ORGANIZATION_BLOCK MAIN:OB1
TITLE= Ciclo Automatico A+/A- per un cilindro a doppio effetto
// Simulatore: 04
// Versione: 1.0
// Data: 28/02/2002
//-------- Descrizione del Controllo --------------------------------
// L'esempio presenta il comando di un cilindro pneumatico a
// doppio effetto (A) mediante un'elettrovalvola 5/2 bistabile (1V1).
// Nel circuito è presente anche un'elettrovalvola del tipo 3/2
// monostabile (0V) che comanda la distribuzione dell'aria nel
// circuito.
// Sulle mandate di alimentazione del cilindro A sono presenti due
// strozzatori unidirezionali per la regolazione della velocità
// delle due corse (A+ e A-) del pistone.
// Un circuito di sicurezza esterno al PLC provvede, quando viene
// disttivato a far rientrare lo stelo del cilindro  nella posizione
// di riposo A- indipendentemente dalle uscite del PLC, che vengono
// resettate quandondo il pulsante SB1 (che simula l'intervento del
// circuito di sicurezza esterno) viene premuto.
// Per le segnalazioni è previste la lampade HL1 che indica
// la presenza dell'aria .
// Agli ingressi del PLC vengono inviati:
// 1)Il selettore SB6 per il comando di 0Y1 che fornisce l'aria
//   compressa al circuito elettropneumatico;
// 2)Il pulsante di arresto a fine ciclo SB3 (NC);
// 3)Il pulsante di inizio ciclo ripetitivo SB2;
// 4)Il pulsante di inizio ciclo non ripetitivo SB4;
// 5)I fine corsa magnetici a0 e a1 che controllano la posizione
//   del pistone rispettivamente in a- e a+;
// L'eventuale mancata eccitazione dell'elettrovalvola distributrice
// non consente l'avvio del ciclo ripetitivo.
//

BEGIN
NETWORK 1 //Comando alimentazione aria elettrovalvola 0V
//
LD I0.0
= Q0.0

NETWORK 2 //Comando Inizio ciclo
//
LD I0.4
O M0.0
A I0.5
A Q0.0
AN I0.3
= M0.0

NETWORK 3 //Comando EV. 1Y1 (uscita cilindro A+)
//
LD M0.0
O I0.6
A I0.1
= Q0.1

NETWORK 4 //Comando EV. 1Y2  (rientro cilindro A-)
//
LD I0.2
= Q0.2

NETWORK 5 //Segnalazione presenza aria compressa
//
LD Q0.0
= Q0.3

END_ORGANIZATION_BLOCK

